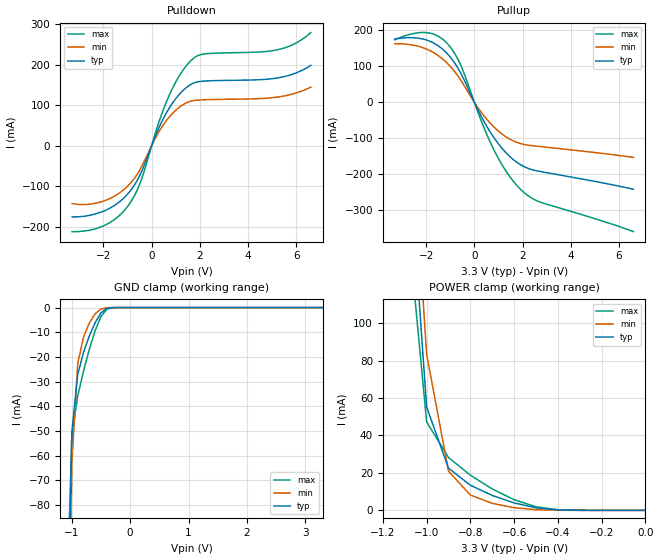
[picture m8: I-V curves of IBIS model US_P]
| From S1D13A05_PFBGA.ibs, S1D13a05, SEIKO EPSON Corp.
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[Model]   US_P
Model_type I/O
Enable Active-Low
Polarity Non-Inverting
Vinh=2.0
Vinl=0.8
C_comp   5p   4p   6p
[Temperature Range] 50   100   0
[Voltage Range]   3.3   3.0   3.6
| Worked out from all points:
|   slope of the pulldown table from 0 to 0.495 V, typ, clamps not added: 7.29 ohm
|   slope of the pullup table from 0 to 0.495 V, typ, clamps not added: 7.69 ohm
|   GND clamp passes 1 mA (typ) near -0.44 V on its own axis
|   POWER clamp passes 1 mA (typ) near -0.47 V on its own axis
[Pullup]
-3.3V     175.6mA    162.7mA    173.3mA
-2.7V     179.5mA    160.3mA    188.2mA
-2V       173.3mA    148.2mA    193.5mA
-1.5V     156.8mA    129.7mA    183.4mA
-1.1V     133.3mA    106.8mA    161.5mA
-600mV    85.25mA    65.06mA    108.2mA
300mV     -40.75mA   -29.06mA   -54.19mA
900mV     -106.4mA   -74.28mA   -143.5mA
1.5V      -152.3mA   -103.3mA   -209.1mA
2.1V      -179.7mA   -117.4mA   -252.6mA
2.8V      -192.8mA   -123.2mA   -278.5mA
6.6V      -241.3mA   -153mA     -358.9mA
[Pulldown]
-3.3V     -175.6mA   -142.6mA   -211.9mA
-1.9V     -159.1mA   -134.5mA   -195mA
-1.3V     -136.7mA   -115.1mA   -170mA
-900mV    -112.4mA   -93.87mA   -141.6mA
-500mV    -74.51mA   -60.57mA   -95.74mA
300mV     43.84mA    34.1mA     57.97mA
700mV     89.74mA    68.6mA     120.2mA
1.2V      129.9mA    96.98mA    177.2mA
1.7V      153.3mA    110.7mA    213.6mA
2.2V      159.3mA    113.3mA    226.2mA
5.3V      167.8mA    120.5mA    237.5mA
6.6V      198mA      144.2mA    278.9mA
[GND Clamp]
-3.3V     -5.502A    -4.83A     -6.436A
-1.1V     -176.1mA   -215.5mA   -132.8mA
-1V       -50.56mA   -63.27mA   -52.18mA
-900mV    -27.23mA   -22.94mA   -36.02mA
-800mV    -18.17mA   -11.94mA   -25.76mA
-700mV    -11.53mA   -6.279mA   -16.89mA
-600mV    -6.084mA   -2.507mA   -9.337mA
-500mV    -2.152mA   -577.5uA   -3.602mA
-400mV    -355.5uA   -75.43uA   -613.8uA
-300mV    -28.44uA   -7.439uA   -35.44uA
3.3V      4.097nA    4.702uA    665.4pA
[POWER Clamp]
-3.3V     5.799A     5.086A     6.768A
-1.1V     221.1mA    263.3mA    170.9mA
-1V       55.2mA     83.29mA    47.21mA
-900mV    22.5mA     20.91mA    28.21mA
-800mV    13.42mA    8.177mA    18.79mA
-700mV    7.949mA    3.747mA    11.4mA
-600mV    3.953mA    1.436mA    5.683mA
-500mV    1.373mA    352.5uA    1.909mA
-400mV    257.6uA    50.87uA    302.8uA
0V        4.097nA    4.463nA    888.1pA
[Ramp]
R_load=50
dV/dt_r   1.719E+0/2.160E-9   1.476E+0/3.238E-9   1.942E+0/1.448E-9
dV/dt_f   1.733E+0/4.838E-9   1.508E+0/8.060E-9   1.955E+0/3.026E-9
